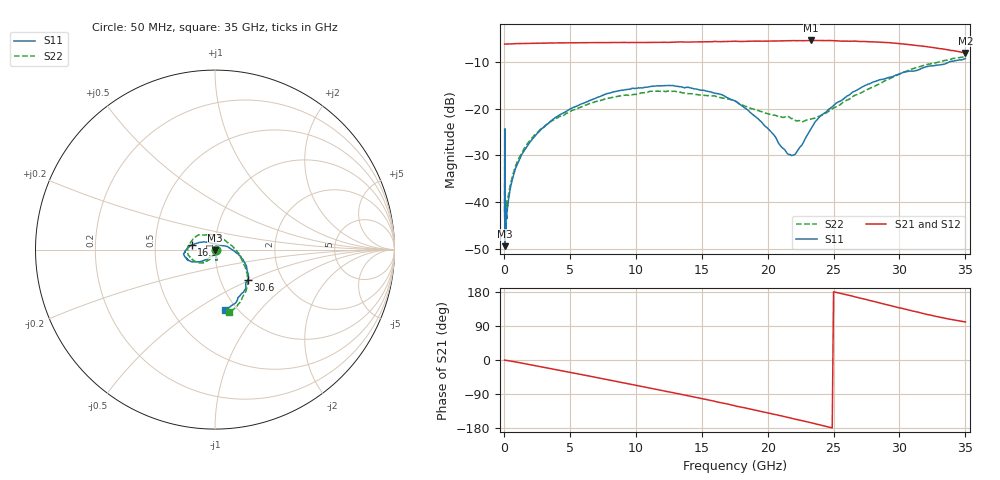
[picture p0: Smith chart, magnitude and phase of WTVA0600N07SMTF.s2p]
! 50 ohm 2-Port S-parameters measured by Modelithics Inc support@modelithics.com  Tampa, FL USA 813-866-6335 (February 2024)
! Smiths Interconnect,  6dB P/N: WTVA0600N07SMTF, Temperature: 25C
! Board: 10 mil Rogers 4350B, Mounting Pad Dimensions: Length: 15 mils, Width: 25 mils, Gap: 40 mils.
# Hz S MA R 50
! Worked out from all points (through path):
!   486 points, 50 MHz to 35 GHz, reference 50 ohm
!   highest |S21| = -5.43 dB at 23.3 GHz (marker M1); lowest = -8.1 dB at 35 GHz (marker M2)
!   group delay of S21, straight-line fit = 20.7 ps
!   lowest |S11| = -49.5 dB at 90 MHz (marker M3), VSWR 1.01, Z = 50.1 - j0.325 ohm
!   |S11| at or under -10 dB: start of sweep to 33.81 GHz
!   |S22| runs from -43.8 to -8.9 dB; largest |S21 - S12| = 0.012
!   S11 on the Smith chart (normalised r, x): 50 MHz: 1.01, -0.01; 16.9 GHz: 0.77, +0.04; 30.6 GHz: 1.34, -0.49; 35 GHz: 0.88, -0.67
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5e7  0.006803 -36.0  0.4892 -0.4  0.4891 -0.3  0.007787 -12.9
8e7  0.006811 -55.0  0.4899 -0.4  0.4896 -0.4  0.008668 -17.0
9e7  0.003362 -75.1  0.4893 -0.5  0.489 -0.5  0.006479 -31.7
1.7e8  0.006726 -76.7  0.4897 -0.9  0.4896 -0.9  0.008476 -53.0
2.5e8  0.008011 -86.1  0.4899 -1.3  0.4899 -1.3  0.009773 -62.2
5e8  0.01441 -98.0  0.4912 -2.8  0.491 -2.7  0.01578 -82.5
1.45e9  0.03399 -115.8  0.4959 -8.7  0.4958 -8.7  0.03513 -105.2
3.3e9  0.06772 -130.4  0.5019 -20.9  0.5019 -20.9  0.0687 -121.0
5.9e9  0.1124 -143.1  0.5063 -38.4  0.5062 -38.4  0.1041 -134.7
8.3e9  0.1506 -154.1  0.5082 -55.0  0.5083 -54.9  0.1323 -151.6
1.17e10  0.1743 -168.8  0.5098 -78.6  0.5097 -78.4  0.1533 -174.5
1.69e10  0.1312 169.2  0.5216 -115.7  0.5216 -115.7  0.1268 143.2
1.76e10  0.1193 164.9  0.5241 -121.7  0.5241 -121.4  0.1185 135.1
1.94e10  0.07448 144.9  0.525 -135.0  0.5247 -134.8  0.0939 118.0
2.17e10  0.03235 86.2  0.5326 -152.8  0.5327 -152.6  0.08001 71.6
2.22e10  0.03409 54.6  0.5316 -156.9  0.5315 -156.5  0.0735 61.5
2.33e10  0.06099 19.1  0.535 -165.7  0.535 -165.4  0.07716 38.0
2.34e10  0.06449 17.0  0.5347 -166.6  0.5349 -166.3  0.07746 36.0
2.65e10  0.1513 -15.8  0.5266 167.8  0.5265 168.3  0.1356 -10.1
2.92e10  0.2157 -33.0  0.5067 144.6  0.5065 145.3  0.2069 -33.5
3.06e10  0.2492 -43.0  0.4854 132.7  0.4856 133.5  0.2539 -43.7
3.5e10  0.343 -80.3  0.3936 100.5  0.3931 100.8  0.358 -77.0
